(* Logix 5000 AddOnInstructionDefinition export AMCI_3202_AOP_Home_CCW; software revision 20.03 *)

ADD_ON_INSTRUCTION AMCI_3202_AOP_Home_CCW   (* revision 1.0, vendor AMCI, ExecuteEnableInFalse *)
VAR_INPUT
   axis_status_bits : INT; {required}
   channel_number : INT; {required}
   Programmed_speed : DINT; {required}
   Acceleration : DINT; {required}
   Deceleration : DINT; {required}
END_VAR
VAR_IN_OUT
   AMCI_3202_output_data : AM:1756_3202:O:0; {required}
END_VAR
VAR_OUTPUT
   EN : BOOL; {access Read Only, visible}
   ER : BOOL; {access Read Only, visible}
END_VAR
VAR
   command_data_block : DINT[8]; {access None}
END_VAR

ROUTINE EnableInFalse   (* ladder *)
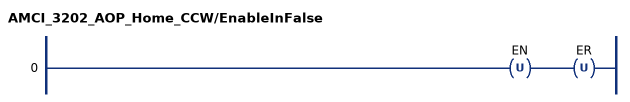
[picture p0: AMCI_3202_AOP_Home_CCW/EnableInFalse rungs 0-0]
   0: OTU(EN)OTU(ER);
END_ROUTINE

ROUTINE Logic   (* ladder *)
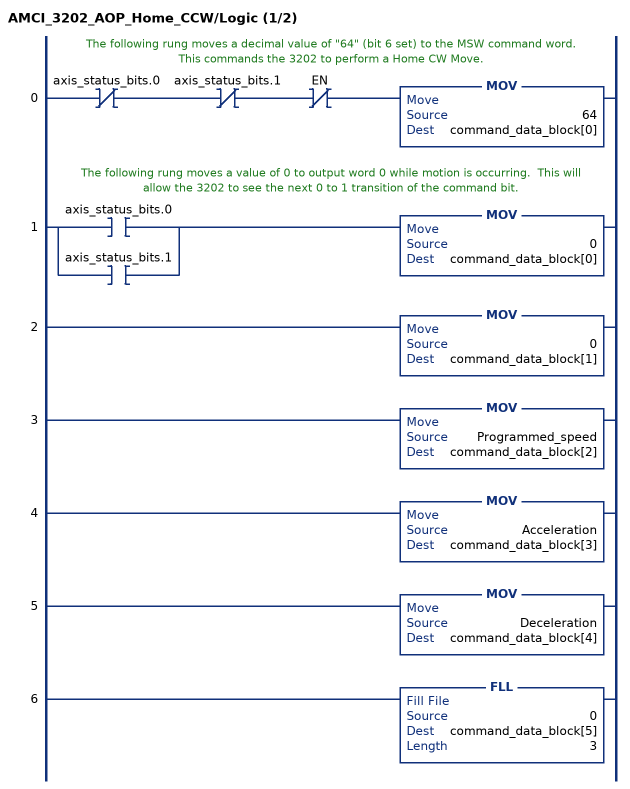
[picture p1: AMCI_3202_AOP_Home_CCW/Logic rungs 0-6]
   // The following rung moves a decimal value of "64" (bit 6 set) to the MSW command word.  This commands the 3202 to perform a Home CW Move.
   0: XIO(axis_status_bits.0)XIO(axis_status_bits.1)XIO(EN)MOV(64,command_data_block[0]);
   // The following rung moves a value of 0 to output word 0 while motion is occurring.  This will allow the 3202 to see the next 0 to 1 transition of the command bit.
   1: [XIC(axis_status_bits.0) ,XIC(axis_status_bits.1) ]MOV(0,command_data_block[0]);
   2: MOV(0,command_data_block[1]);
   3: MOV(Programmed_speed,command_data_block[2]);
   4: MOV(Acceleration,command_data_block[3]);
   5: MOV(Deceleration,command_data_block[4]);
   6: FLL(0,command_data_block[5],3);
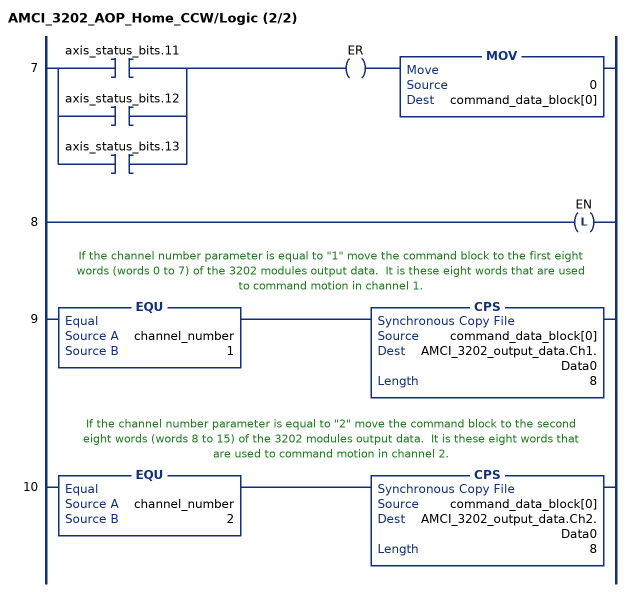
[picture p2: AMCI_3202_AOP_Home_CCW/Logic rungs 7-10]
   7: [XIC(axis_status_bits.11) ,XIC(axis_status_bits.12) ,XIC(axis_status_bits.13) ]OTE(ER)MOV(0,command_data_block[0]);
   8: OTL(EN);
   // If the channel number parameter is equal to "1" move the command block to the first eight words (words 0 to 7) of the 3202 modules output data.  It is these eight words that are used to command motion in channel 1.
   9: EQU(channel_number,1)CPS(command_data_block[0],AMCI_3202_output_data.Ch1.Data0,8);
   // If the channel number parameter is equal to "2" move the command block to the second eight words (words 8 to 15) of the 3202 modules output data.  It is these eight words that are used to command motion in channel 2.
   10: EQU(channel_number,2)CPS(command_data_block[0],AMCI_3202_output_data.Ch2.Data0,8);
END_ROUTINE
END_ADD_ON_INSTRUCTION
